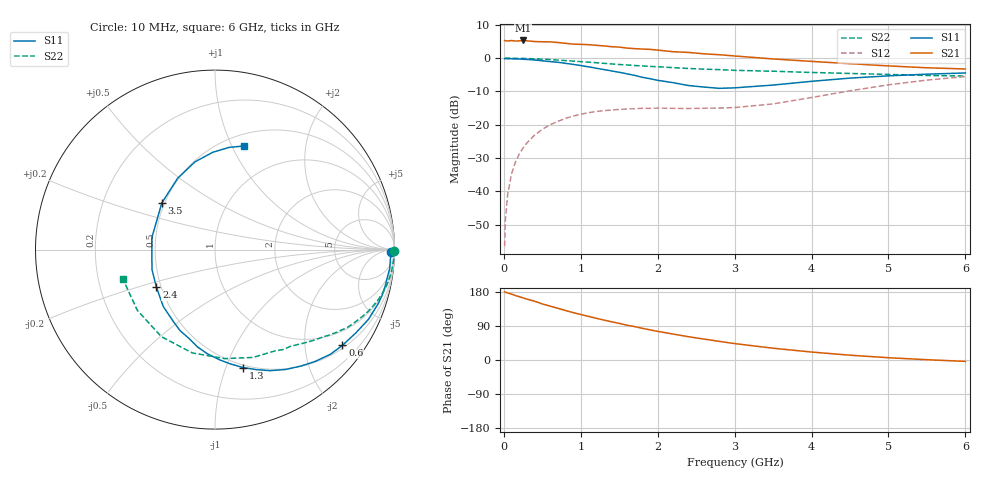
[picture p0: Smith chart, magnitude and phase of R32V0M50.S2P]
! SIEMENS Small Signal Semiconductors
! BFR181
! Si NPN RF Bipolar Junction Transistor in SOT23
! VCE = 2 V  IC = 0.5 mA
! Common Emitter S-Parameters:  May  1996
# GHz  S  MA  R  50
!  f  S11  S21  S12  S22
! GHz  MAG  ANG  MAG  ANG  MAG  ANG  MAG  ANG
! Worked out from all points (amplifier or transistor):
!   36 points, 10 MHz to 6 GHz, reference 50 ohm
!   highest |S21| = 5.3 dB at 250 MHz (marker M1)
!   |S21| within 3 dB of that: start of sweep to 2.043 GHz
!   unconditionally stable (mu >= 1): 2.347 GHz to 3.97 GHz
!   at 250 MHz: K = 0.12, MSG = 16.1 dB, |S12| = -27.0 dB
!   at 1.4 GHz: K = 0.62, MSG = 9.5 dB, |S12| = -15.6 dB
!   at 6 GHz: K = 0.93, MSG = 1.1 dB, |S12| = -5.5 dB
!   S11 on the Smith chart (normalised r, x): 10 MHz: 71, -42; 600 MHz: 0.57, -2.90; 1.3 GHz: 0.48, -1.15; 2.4 GHz: 0.47, -0.23; 3.5 GHz: 0.48, +0.30; 6 GHz: 0.62, +1.11
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0.01  0.9794 -0.7  1.834 179.8  0.0015 94.5  0.9999 -0.3
0.02  0.981 -1.3  1.829 178.7  0.0037 85.0  0.9973 -0.7
0.05  0.9786 -3.0  1.812 177.0  0.009 89.3  0.9986 -1.5
0.1  0.9793 -6.2  1.838 173.9  0.0183 86.4  0.9978 -2.9
0.15  0.9731 -8.9  1.812 170.1  0.0272 83.5  0.9948 -4.5
0.25  0.965 -15.5  1.845 163.9  0.0448 79.2  0.9909 -7.3
0.4  0.9393 -24.4  1.776 155.2  0.0698 73.1  0.9781 -11.5
0.5  0.9123 -30.5  1.763 147.9  0.0854 68.8  0.9658 -14.3
0.6  0.8882 -36.9  1.758 142.3  0.0997 64.9  0.9518 -17.0
0.8  0.8367 -48.1  1.672 130.7  0.1245 57.6  0.9198 -22.0
1.1  0.7412 -65.5  1.596 115.1  0.1517 48.6  0.8715 -28.4
1.3  0.675 -76.7  1.529 105.5  0.163 43.4  0.8363 -32.3
1.5  0.6142 -87.7  1.467 96.6  0.1695 39.4  0.803 -35.8
1.8  0.5158 -106.3  1.37 83.6  0.1768 35.4  0.7651 -40.1
2.2  0.4287 -132.2  1.25 68.5  0.1763 32.9  0.7205 -46.2
2.4  0.388 -147.2  1.219 61.4  0.1755 33.5  0.7005 -49.1
3  0.3582 169.3  1.079 43.3  0.1812 39.5  0.6565 -59.2
3.5  0.3943 138.7  0.973 31.1  0.2054 46.0  0.637 -70.6
4.5  0.5015 102.8  0.826 12.7  0.3234 49.0  0.5894 -102.4
5  0.5424 91.3  0.765 6.0  0.3979 43.9  0.5696 -121.7
5.5  0.5751 82.1  0.717 0.8  0.4682 36.3  0.5492 -142.0
6  0.5993 74.4  0.688 -3.7  0.5296 27.6  0.5389 -162.4
